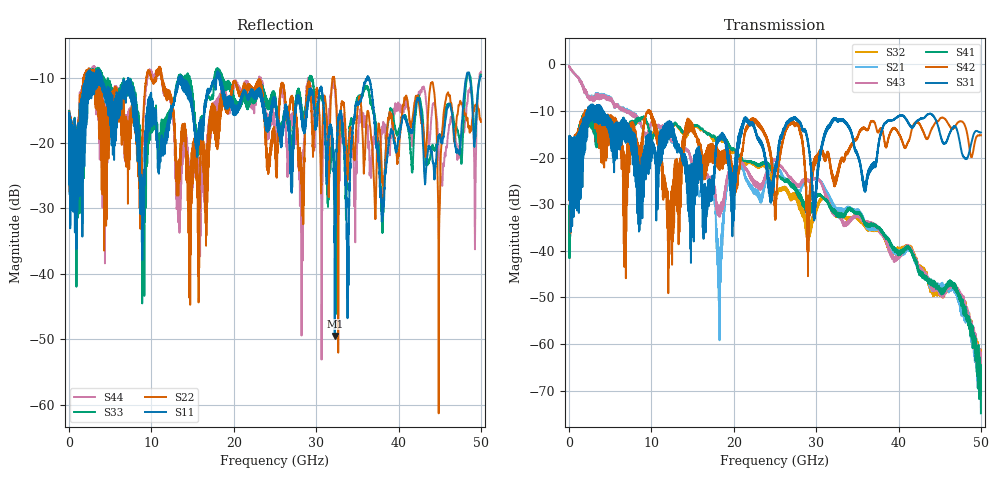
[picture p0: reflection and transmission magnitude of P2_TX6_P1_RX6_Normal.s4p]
!Keysight Technologies,N5225A,MY51441389,A.10.49.11
!Date: Monday, July 08, 2019 14:58:21
!Correction: S11(Full 4 Port(1,2,3,4))
!S12(Full 4 Port(1,2,3,4))
!S13(Full 4 Port(1,2,3,4))
!S14(Full 4 Port(1,2,3,4))
!S21(Full 4 Port(1,2,3,4))
!S22(Full 4 Port(1,2,3,4))
!S23(Full 4 Port(1,2,3,4))
!S24(Full 4 Port(1,2,3,4))
!S31(Full 4 Port(1,2,3,4))
!S32(Full 4 Port(1,2,3,4))
!S33(Full 4 Port(1,2,3,4))
!S34(Full 4 Port(1,2,3,4))
!S41(Full 4 Port(1,2,3,4))
!S42(Full 4 Port(1,2,3,4))
!S43(Full 4 Port(1,2,3,4))
!S44(Full 4 Port(1,2,3,4))
!S4P File: Measurements: <S11,S12,S13,S14>,
!<S21,S22,S23,S24>,
!<S31,S32,S33,S34>,
!<S41,S42,S43,S44>:
# Hz S  dB  R 50
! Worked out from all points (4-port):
!   5000 points, 10 MHz to 50 GHz, reference 50 ohm
!   strongest paths, dB at 10 MHz, 12.51 GHz, 25.01 GHz, 37.51 GHz, 50 GHz:
!     S31: -19.1, -15.2, -22.9, -18.4, -14.6
!     S42: -19.0, -43.0, -30.8, -14.6, -15.2
!     S41: -33.6, -12.8, -23.8, -34.9, -74.9
!     S43: -0.4, -16.6, -20.4, -35.0, -62.7
!     S21: -0.4, -16.9, -21.4, -35.1, -68.1
!     S32: -32.8, -12.8, -27.6, -35.4, -65.3
!   lowest |S11| = -49.5 dB at 32.26 GHz (marker M1), VSWR 1.01, Z = 49.9 + j0.327 ohm
!   |S11| at or under -10 dB: 3.955 GHz to 13.33 GHz (9.373 GHz wide, 108 % of centre); 18.33 GHz to 36.21 GHz (17.88 GHz wide, 65.6 % of centre); 36.37 GHz to 48.22 GHz (11.85 GHz wide, 28 % of centre)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
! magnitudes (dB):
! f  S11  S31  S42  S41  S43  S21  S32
! 10 MHz  -17.8  -19.1  -19.0  -33.6  -0.4  -0.4  -32.8
! 1.87 GHz  -14.7  -14.4  -11.3  -10.6  -5.8  -5.8  -11.3
! 9.01 GHz  -32.3  -23.3  -15.0  -11.3  -14.5  -14.5  -11.7
! 18.22 GHz  -10.1  -15.8  -18.9  -15.6  -32.7  -51.8  -15.9
! 20.56 GHz  -14.2  -18.1  -23.6  -19.4  -20.7  -21.9  -20.0
! 32.26 GHz  -49.5  -11.6  -24.9  -32.0  -32.5  -31.1  -32.3
! 50 GHz  -9.8  -14.6  -15.2  -74.9  -62.7  -68.1  -65.3
